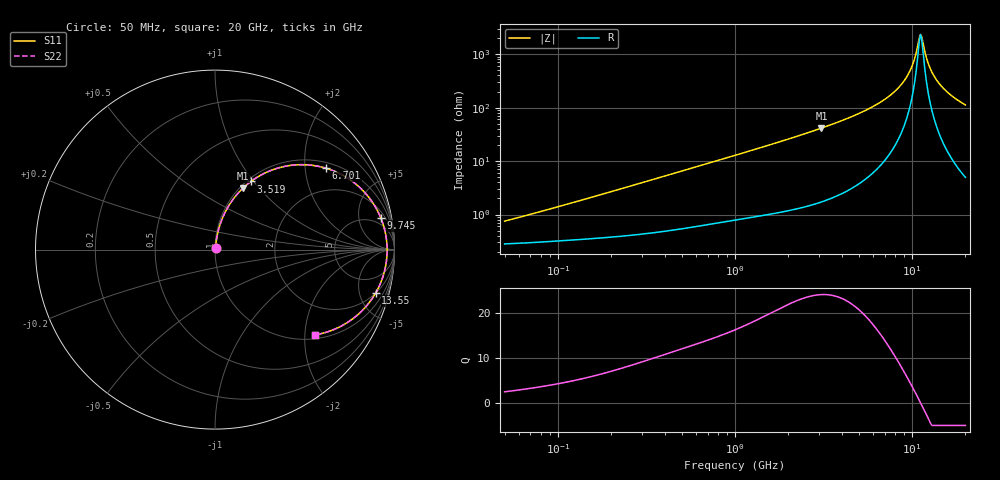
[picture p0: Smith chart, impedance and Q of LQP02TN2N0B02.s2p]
!Murata Part Number: LQP02TN2N0B02
!These Parameters are Measured in Series Mode Connection
!  o--[Z]--o
!Port1  Port2
!  o-------o
!Freq. Start=50[MHz] Stop=20[GHz], 401[Steps]
# Hz S RI R 50
!Freq.(Hz) S11(Real) S11(Imag) S21(Real) S21(Imag) S12(Real) S12(Imag) S22(Real) S22(Imag)
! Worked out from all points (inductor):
!   401 points, 50 MHz to 20 GHz, reference 50 ohm
!   read as one part in series: L = 2.18 nH near 63.54 MHz
!   highest Q = 24 at 3.075 GHz (marker M1), where L = 2.14 nH
!   self-resonance near 11.15 GHz
!   S11 on the Smith chart (normalised r, x): 50 MHz: 1.01, +0.01; 3.519 GHz: 1.04, +0.97; 6.701 GHz: 1.17, +2.58; 9.745 GHz: 3, +10; 13.55 GHz: 2.03, -6.99; 20 GHz: 1.10, -2.24
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5e7  0.00286 0.00693  0.9971 -0.00693  0.9971 -0.00693  0.00286 0.00693
1.364002e8  0.00375 0.0182  0.9963 -0.0182  0.9963 -0.0182  0.00375 0.0182
3.721004e8  0.007 0.048  0.993 -0.048  0.993 -0.048  0.007 0.048
1e9  0.0235 0.1237  0.9765 -0.1237  0.9765 -0.1237  0.0235 0.1237
1.793498e9  0.0595 0.2139  0.9405 -0.2139  0.9405 -0.2139  0.0595 0.2139
2.728004e9  0.1251 0.3105  0.8749 -0.3105  0.8749 -0.3105  0.1251 0.3105
3.075291e9  0.1559 0.3426  0.8441 -0.3426  0.8441 -0.3426  0.1559 0.3426
3.519108e9  0.2 0.3796  0.8 -0.3796  0.8 -0.3796  0.2 0.3796
4.89267e9  0.3658 0.4585  0.6342 -0.4585  0.6342 -0.4585  0.3658 0.4585
6.701223e9  0.6181 0.4536  0.3819 -0.4536  0.3819 -0.4536  0.6181 0.4536
7.442007e9  0.716 0.4123  0.284 -0.4123  0.284 -0.4123  0.716 0.4123
8.644534e9  0.8469 0.3039  0.1531 -0.3039  0.1531 -0.3039  0.8469 0.3039
9.745021e9  0.9241 0.1758  0.0759 -0.1758  0.0759 -0.1758  0.9241 0.1758
1.019291e10  0.9427 0.1204  0.0573 -0.1204  0.0573 -0.1204  0.9427 0.1204
1.098561e10  0.9583 0.0228  0.0417 -0.0228  0.0417 -0.0228  0.9583 0.0228
1.115139e10  0.959 0.00288  0.041 -0.00288  0.041 -0.00288  0.959 0.00288
1.149051e10  0.9578 -0.0369  0.0422 0.0369  0.0422 0.0369  0.9578 -0.0369
1.201863e10  0.9499 -0.096  0.0501 0.096  0.0501 0.096  0.9499 -0.096
1.257102e10  0.9349 -0.1531  0.0651 0.1531  0.0651 0.1531  0.9349 -0.1531
1.354865e10  0.8956 -0.241  0.1044 0.241  0.1044 0.241  0.8956 -0.241
1.597544e10  0.7645 -0.3879  0.2355 0.3879  0.2355 0.3879  0.7645 -0.3879
2e10  0.5551 -0.4754  0.4449 0.4754  0.4449 0.4754  0.5551 -0.4754
